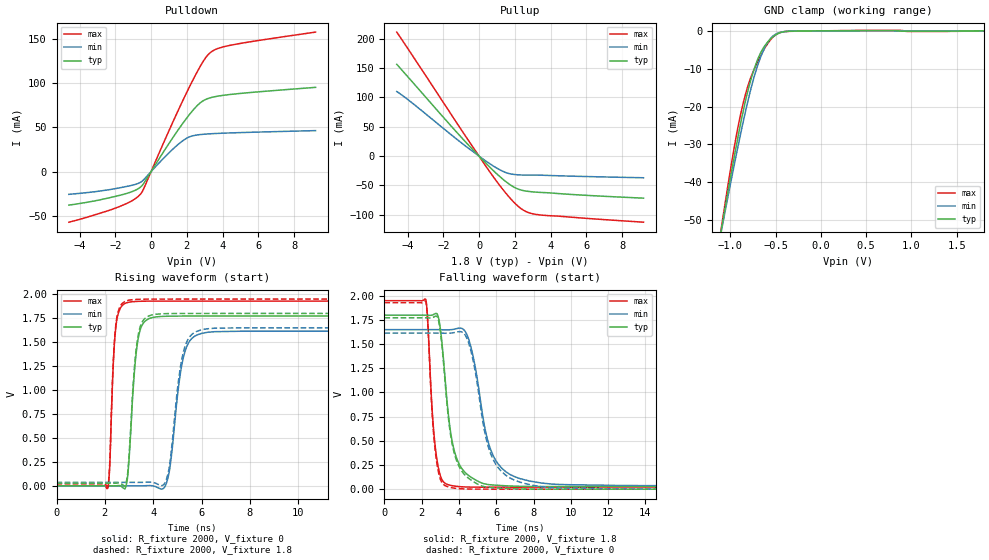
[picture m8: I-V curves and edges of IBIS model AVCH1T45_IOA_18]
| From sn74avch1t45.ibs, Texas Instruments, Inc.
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[Model]   AVCH1T45_IOA_18
Model_type  I/O
Vinl=0.5775
Vinh=1.2675
Enable   Active-Low
Vref =   0
Rref =   2000
Cref =   15p
Vmeas =   0.9
| variable   typ   min   max
C_comp   5.27pF   4.50pF   5.87pF
| C_pullup   4.78pF   3.53pF   6.89pF
| C_pulldown   4.68pF   4.09pF   5.05pF
| C_tri-state   5.27pF   4.50pF   5.87pF
[Temperature Range]   40   100   -40
| Ambient temperature   25   85   -40
[Voltage range]   1.8   1.65   1.95
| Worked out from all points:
|   slope of the pulldown table from 0 to 0.27 V, typ, clamps not added: 30.8 ohm
|   slope of the pullup table from 0 to 0.27 V, typ, clamps not added: 31.4 ohm
|   GND clamp passes 1 mA (typ) near -0.49 V on its own axis
|   rising waveform, R_fixture 2000, V_fixture 0: 20-80 % time 290ps typ, 449ps min, 186ps max; typ from 0 V to 1.77 V
|   falling waveform, R_fixture 2000, V_fixture 1.8: 20-80 % time 651ps typ, 999ps min, 375ps max; typ from 1.8 V to 0.027 V
|   rising waveform, R_fixture 2000, V_fixture 1.8: 20-80 % time 288ps typ, 441ps min, 184ps max; typ from 0.027 V to 1.8 V
|   falling waveform, R_fixture 2000, V_fixture 0: 20-80 % time 653ps typ, 998ps min, 362ps max; typ from 1.77 V to 0 V
[GND Clamp]
| AVCH1T45_IOA_18
|   Voltage   I(typ)   I(min)   I(max)
-4.6V     -599.6mA   -548.2mA   -664.6mA
-1.1V     -52.38mA   -52.81mA   -51.88mA
-1.075V   -48.92mA   -49.68mA   -47.98mA
-930mV    -29.69mA   -32.08mA   -27.04mA
-830mV    -18.1mA    -20.91mA   -16.44mA
-755mV    -11.37mA   -13.59mA   -11.08mA
-675mV    -6.227mA   -7.502mA   -6.966mA
-595mV    -3.153mA   -3.319mA   -3.603mA
-520mV    -1.409mA   -1.191mA   -1.426mA
-440mV    -417.5uA   -333.3uA   -376.2uA
-275mV    -54.37uA   -36.84uA   -89.06uA
1.8V      918.7pA    21.47uA    -48.34uA
[Pulldown]
| AVCH1T45_IOA_18
|   Voltage   I(typ)   I(min)   I(max)
-4.6V     -37.94mA   -25.73mA   -57.23mA
-1.8V     -27.09mA   -18.52mA   -39.79mA
-1.045V   -22.5mA    -15.36mA   -32.7mA
-590mV    -17.44mA   -12.06mA   -25.35mA
-395mV    -12.81mA   -8.801mA   -18.52mA
1.005V    31.93mA    21.31mA    46.48mA
1.825V    55.97mA    35.61mA    82.46mA
2.68V     76.51mA    41.68mA    116.5mA
3.05V     81.53mA    42.39mA    128.7mA
3.34V     83.6mA     42.77mA    135mA
4.585V    87.54mA    43.82mA    143.4mA
9.2V      95.24mA    46.32mA    157.7mA
[Pullup]
| AVCH1T45_IOA_18
|   Voltage   I(typ)   I(min)   I(max)
-4.6V     156.3mA    109.9mA    211.2mA
-3.695V   125.1mA    89.45mA    169.9mA
-1.245V   40.55mA    28.8mA     56.51mA
535mV     -16.77mA   -11.6mA    -23.84mA
1.065V    -32.16mA   -21.66mA   -46.14mA
1.49V     -43.16mA   -27.88mA   -62.67mA
1.925V    -52.28mA   -31.05mA   -77.72mA
2.305V    -57.27mA   -32.09mA   -88.3mA
2.77V     -60.1mA    -32.26mA   -96.25mA
3.4V      -61.74mA   -32.39mA   -100.1mA
9.2V      -71.58mA   -36.85mA   -112.5mA
[Ramp]
| AVCH1T45_IOA_18
| variable   typ   min   max
dV/dt_r   1.08/3.02E-10   0.99/4.61E-10   1.17/1.95E-10
dV/dt_f   1.07/6.57E-10   0.98/1.01E-09   1.17/3.80E-10
R_load = 2000
[Rising Waveform]
| AVCH1T45_IOA_18
R_fixture =   2000
C_fixture =   0
L_fixture =   0
V_fixture =   0
V_fixture_min = 0
V_fixture_max = 0
|   Time   V(typ)   V(min)   V(max)
0s        21.35nV    98.25nV    665.6pV
2.13ns    39.11uV    -109.1nV   -19.45mV
2.455ns   606.1uV    -20.46uV   1.659V
2.945ns   104.7mV    15.91uV    1.914V
3.36ns    1.509V     -172.9uV   1.926V
3.965ns   1.757V     994.9uV    1.929V
4.555ns   1.77V      32.36mV    1.929V
5.245ns   1.772V     1.336V     1.929V
6.025ns   1.773V     1.593V     1.929V
29.99ns   1.773V     1.615V     1.929V
[Falling Waveform]
| AVCH1T45_IOA_18
R_fixture =   2000
C_fixture =   0
L_fixture =   0
V_fixture =   1.8
V_fixture_min = 1.65
V_fixture_max = 1.95
|   Time   V(typ)   V(min)   V(max)
0s        1.8V       1.65V      1.95V
2.215ns   1.8V       1.65V      1.964V
2.745ns   1.817V     1.65V      407.2mV
3.015ns   1.636V     1.649V     131mV
3.41ns    805.8mV    1.648V     46.68mV
3.76ns    388.6mV    1.656V     32.07mV
4.295ns   179.1mV    1.641V     23.26mV
5.7ns     45.05mV    407.7mV    20.42mV
7.26ns    29.59mV    109.7mV    20.34mV
29.99ns   27.01mV    36.05mV    20.32mV
[Rising Waveform]
| AVCH1T45_IOA_18
R_fixture =   2000
C_fixture =   0
L_fixture =   0
V_fixture =   1.8
V_fixture_min = 1.65
V_fixture_max = 1.95
|   Time   V(typ)   V(min)   V(max)
0s        27.01mV    36.05mV    20.32mV
2.13ns    27.05mV    36.05mV    1.142mV
2.45ns    27.53mV    36.03mV    1.673V
2.945ns   135.6mV    36.06mV    1.936V
3.35ns    1.53V      35.88mV    1.947V
3.94ns    1.784V     37.75mV    1.95V
4.55ns    1.798V     69.07mV    1.95V
5.23ns    1.8V       1.377V     1.95V
6.005ns   1.8V       1.63V      1.95V
29.99ns   1.8V       1.65V      1.95V
[Falling Waveform]
| AVCH1T45_IOA_18
R_fixture =   2000
C_fixture =   0
L_fixture =   0
V_fixture =   0
V_fixture_min = 0
V_fixture_max = 0
|   Time   V(typ)   V(min)   V(max)
0s        1.773V     1.615V     1.929V
2.215ns   1.773V     1.615V     1.943V
2.74ns    1.79V      1.615V     372.4mV
3ns       1.629V     1.614V     102.8mV
3.385ns   822.3mV    1.613V     25.67mV
3.74ns    376mV      1.619V     10.89mV
4.285ns   153.8mV    1.606V     2.569mV
5.69ns    17.29mV    370.9mV    86.55uV
7.28ns    2.194mV    71.85mV    11.43uV
29.99ns   89.6nV     1.395uV    173.5nV
